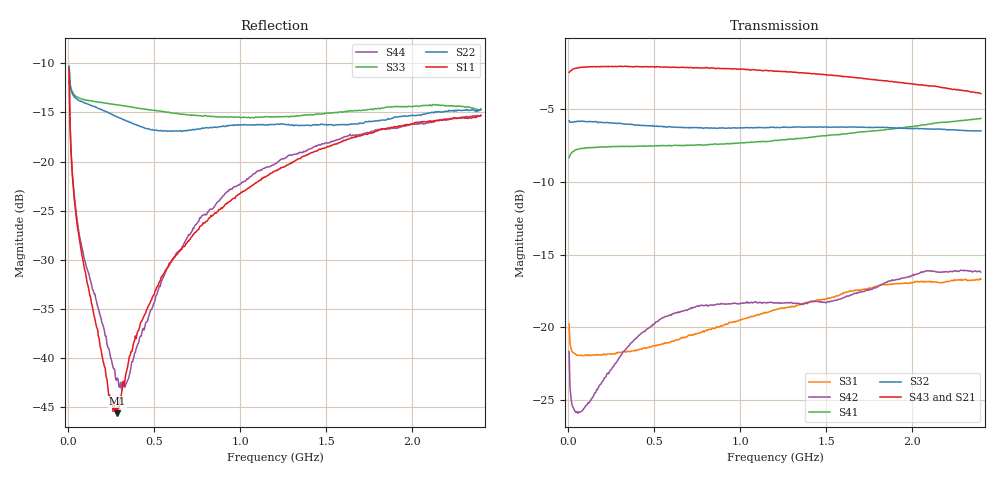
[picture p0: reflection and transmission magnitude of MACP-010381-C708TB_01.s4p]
!Agilent Technologies,E5071B,JP1KK00267,A.09.10
!Date: Mon Mar 23 10:56:30 2020
!DD.  Test Board PCB PT-0014848.  Pin Port mapping: Port1 – pin1, Port1 – pin2, Port3 – pin4, Port4 – pin5
!Data & Calibration Information:
!Freq	S11:SOLT4(ON)	S12:SOLT4(ON)	S13:SOLT4(ON)	S14:SOLT4(ON)
!	S21:SOLT4(ON)	S22:SOLT4(ON)	S23:SOLT4(ON)	S24:SOLT4(ON)
!	S31:SOLT4(ON)	S32:SOLT4(ON)	S33:SOLT4(ON)	S34:SOLT4(ON)
!	S41:SOLT4(ON)	S42:SOLT4(ON)	S43:SOLT4(ON)	S44:SOLT4(ON)
# Hz S MA R 75
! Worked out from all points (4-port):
!   480 points, 5 MHz to 2.4 GHz, reference 75 ohm
!   strongest paths, dB at 5 MHz, 605 MHz, 1.205 GHz, 1.805 GHz, 2.4 GHz:
!     S43: -2.5, -2.1, -2.4, -3.0, -3.9
!     S21: -2.5, -2.2, -2.5, -3.0, -4.0
!     S32: -5.8, -6.2, -6.3, -6.2, -6.5
!     S41: -8.3, -7.5, -7.1, -6.5, -5.6
!     S42: -21.7, -19.1, -18.3, -17.1, -16.2
!     S31: -19.8, -20.9, -18.8, -17.1, -16.7
!   lowest |S11| = -45.6 dB at 285 MHz (marker M1), VSWR 1.01, Z = 74.3 - j0.392 ohm
!   |S11| at or under -10 dB: start of sweep to end of sweep
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5000000  0.2965 111.1  0.7442 15.1  0.08079 153.1  0.3857 25.1
         0.7468 15.1  0.3049 144.3  0.5115 -172.4  0.09789 163.3
         0.1028 165.8  0.5134 -172.2  0.3055 145.4  0.7539 14.9
         0.3829 25.3  0.08266 153.9  0.752 14.9  0.2942 112.1
2.5e7  0.08264 116.6  0.7626 3.3  0.05367 166.3  0.4032 6.2
       0.7664 3.1  0.2202 166.1  0.5086 -179.9  0.07679 172.3
       0.08221 172.5  0.5076 -179.9  0.2253 167.4  0.7738 3.1
       0.4015 6.2  0.05363 169.3  0.7701 3.0  0.08415 120.1
6.5e7  0.03996 118.6  0.7723 -0.1  0.04983 168.0  0.4128 2.7
       0.7754 -0.2  0.2039 169.1  0.5097 176.1  0.07446 172.5
       0.08016 172.0  0.511 175.9  0.2104 171.7  0.7829 -0.1
       0.4102 2.7  0.05096 178.0  0.7815 -0.1  0.04195 124.6
2.85e8  0.005247 -149.9  0.7821 -8.5  0.05404 150.9  0.4203 -1.6
        0.7826 -8.5  0.1685 163.5  0.5054 159.7  0.07866 157.6
        0.08161 156.0  0.5015 158.8  0.1944 170.5  0.7887 -8.4
        0.4178 -1.3  0.07651 176.5  0.7877 -8.4  0.007943 -178.9
5.5e8  0.02639 -88.2  0.7811 -17.5  0.06753 127.9  0.4211 -4.3
       0.7808 -17.5  0.1431 166.6  0.4967 141.5  0.08936 138.3
       0.08765 136.1  0.4905 140.6  0.1799 167.1  0.7863 -17.2
       0.4219 -4.0  0.108 145.2  0.7843 -17.0  0.02562 -86.5
9.2e8  0.06141 -89.8  0.768 -30.1  0.09303 101.2  0.428 -6.9
       0.7713 -29.9  0.152 168.5  0.4896 117.0  0.1114 111.7
       0.1023 110.1  0.4837 116.8  0.1682 164.9  0.7756 -29.3
       0.4273 -7.0  0.1206 105.3  0.7748 -29.0  0.06955 -86.1
2.4e9  0.172 -127.0  0.6284 -81.6  0.1534 20.9  0.5177 -24.4
       0.6294 -81.9  0.1831 133.7  0.4749 22.3  0.1491 18.7
       0.1462 18.8  0.4738 22.9  0.1856 124.9  0.637 -78.3
       0.5228 -24.6  0.1548 20.7  0.636 -78.6  0.1711 -118.7
